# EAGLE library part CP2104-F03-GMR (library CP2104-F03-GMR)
USB-to-UART 1-CH 576byte FIFO 3.3V Automotive 24-Pin QFN EP T/R Source: Datasheet
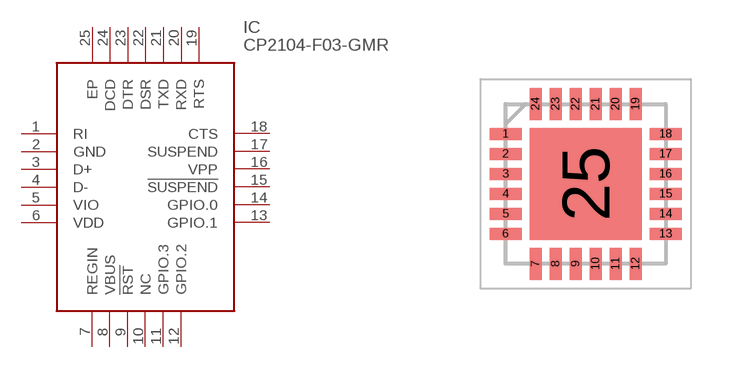
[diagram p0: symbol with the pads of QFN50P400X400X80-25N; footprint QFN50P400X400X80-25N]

Designator prefix IC

## CP2104-F03-GMR (Description: USB-to-UART 1-CH 576byte FIFO 3.3V Automotive 24-Pin QFN EP T/R; Height: 0.8mm; Manufacturer_Name: Silicon Labs; Manufacturer_Part_Number: CP2104-F03-GMR; Mouser_Part_Number: 634-CP2104-F03-GMR; Mouser_Price-Stock: https://www.mouser.co.uk/ProductDetail/Silicon-Labs/CP2104-F03-GMR?qs=1CB38rTTsYrRJKVkczeRzA%3D%3D)  [QFN50P400X400X80-25N]
1  RI
2  GND
3  D+
4  D-
5  VIO
6  VDD
7  REGIN
8  VBUS
9  !RST
10  NC  nc
11  GPIO.3
12  GPIO.2
13  GPIO.1
14  GPIO.0
15  !SUSPEND
16  VPP
17  SUSPEND
18  CTS
19  RTS
20  RXD
21  TXD
22  DSR
23  DTR
24  DCD
25  EP

## Footprint QFN50P400X400X80-25N (pad centres in mm)
QFN-24 (4x4 mm)
smd 0.8 x 0.3: 1 -2,1.25; 2 -2,0.75; 3 -2,0.25; 4 -2,-0.25; 5 -2,-0.75; 6 -2,-1.25; 13 2,-1.25; 14 2,-0.75; 15 2,-0.25; 16 2,0.25; 17 2,0.75; 18 2,1.25
smd 0.3 x 0.8: 7 -1.25,-2; 8 -0.75,-2; 9 -0.25,-2; 10 0.25,-2; 11 0.75,-2; 12 1.25,-2; 19 1.25,2; 20 0.75,2; 21 0.25,2; 22 -0.25,2; 23 -0.75,2; 24 -1.25,2
smd 2.8 x 2.8: 25 0,0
